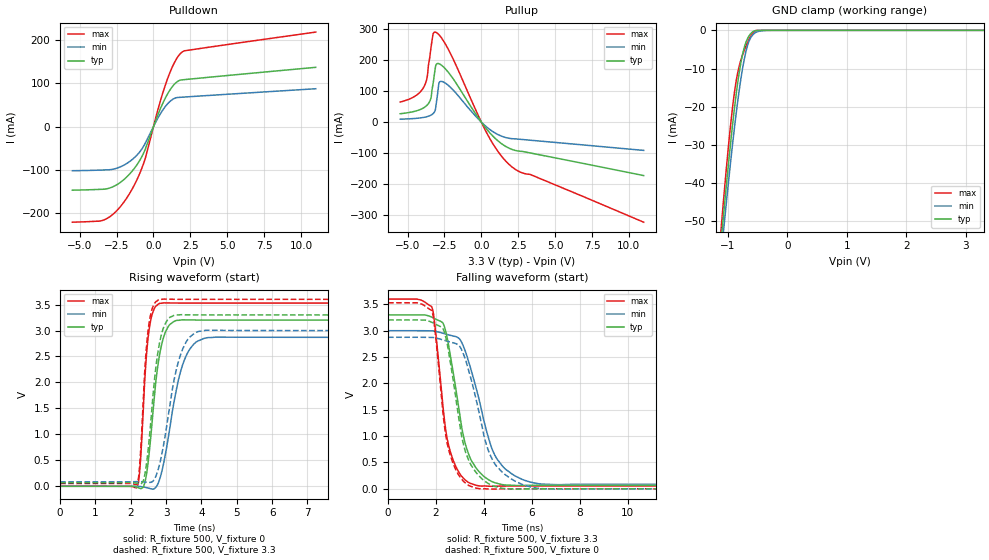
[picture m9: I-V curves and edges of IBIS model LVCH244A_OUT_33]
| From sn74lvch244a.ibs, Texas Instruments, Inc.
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[Model]   LVCH244A_OUT_33
Model_type  3-state
Enable   Active-Low
Vref =   0
Rref =   500
Cref =   50p
Vmeas =   1.5
| variable   typ   min   max
C_comp   4.99pF   4.68pF   5.36pF
| C_pullup   6.79pF   5.44pF   7.57pF
| C_pulldown   5.99pF   4.56pF   7.14pF
| C_tri-state   4.99pF   4.68pF   5.36pF
[Temperature Range]   40   100   -40
| Ambient temperature   25   85   -40
[Voltage range]   3.3   3   3.6
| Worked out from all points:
|   slope of the pulldown table from 0 to 0.495 V, typ, clamps not added: 11.4 ohm
|   slope of the pullup table from 0 to 0.495 V, typ, clamps not added: 16.4 ohm
|   GND clamp passes 1 mA (typ) near -0.62 V on its own axis
|   rising waveform, R_fixture 500, V_fixture 0: 20-80 % time 302ps typ, 479ps min, 190ps max; typ from 0 V to 3.2 V
|   falling waveform, R_fixture 500, V_fixture 3.3: 20-80 % time 767ps typ, 1.07ns min, 558ps max; typ from 3.3 V to 0.068 V
|   rising waveform, R_fixture 500, V_fixture 3.3: 20-80 % time 292ps typ, 464ps min, 185ps max; typ from 0.068 V to 3.3 V
|   falling waveform, R_fixture 500, V_fixture 0: 20-80 % time 739ps typ, 1ns min, 551ps max; typ from 3.2 V to 0 V
[GND Clamp]
| LVCH244A_OUT_33
|   Voltage   I(typ)   I(min)   I(max)
-5.5V     -943.7mA   -897.4mA   -1.02A
-1.13V    -57.95mA   -61.61mA   -54.83mA
-1.1V     -52.83mA   -56.76mA   -49.28mA
-1.075V   -48.62mA   -52.78mA   -44.76mA
-1.05V    -44.49mA   -48.86mA   -40.33mA
-945mV    -28.12mA   -33.13mA   -23.39mA
-845mV    -14.88mA   -19.82mA   -11.9mA
-770mV    -7.53mA    -11.54mA   -7.224mA
-700mV    -3.298mA   -5.769mA   -4.298mA
-630mV    -1.124mA   -2.323mA   -1.902mA
-550mV    -125.2uA   -727.7uA   -227uA
3.3V      1.171nA    103.7nA    -1.528nA
[Pulldown]
| LVCH244A_OUT_33
|   Voltage   I(typ)   I(min)   I(max)
-5.5V     -146.4mA   -101.6mA   -220.3mA
-3.715V   -144.7mA   -100.3mA   -217.9mA
-3.27V    -143.9mA   -99.76mA   -213.7mA
-2.52V    -134.6mA   -96.13mA   -194.9mA
-1.76V    -114.3mA   -83.77mA   -161.9mA
-1.14V    -88.83mA   -66.3mA    -123.8mA
-625mV    -57.63mA   -42.51mA   -80.68mA
390mV     34.91mA    25.18mA    49.89mA
1.01V     78.63mA    54.56mA    115.5mA
1.49V     100.2mA    66.1mA     152mA
1.93V     107.9mA    67.88mA    171.6mA
11V       136.8mA    87.39mA    218mA
[Pullup]
| LVCH244A_OUT_33
|   Voltage   I(typ)   I(min)   I(max)
-5.5V     27.15mA    9.676mA    64.84mA
-4.47V    35.52mA    12.08mA    84.48mA
-3.88V    47.09mA    15.63mA    115mA
-3.675V   55mA       17.9mA     145.1mA
-3.43V    75.88mA    22.33mA    234.3mA
-3.27V    125.3mA    27.62mA    284.1mA
-3.065V   185.7mA    57.97mA    288.8mA
-2.875V   188mA      125.7mA    281.3mA
-2.57V    177.9mA    129.2mA    261.6mA
385mV     -24.04mA   -16.62mA   -36.62mA
1.895V    -84.17mA   -52.11mA   -136.8mA
11V       -171.9mA   -90.86mA   -321.9mA
[Ramp]
| LVCH244A_OUT_33
| variable   typ   min   max
dV/dt_r   1.95/3.12E-10   1.76/5.01E-10   2.14/1.97E-10
dV/dt_f   1.94/7.68E-10   1.75/1.10E-09   2.13/5.60E-10
R_load = 500
[Rising Waveform]
| LVCH244A_OUT_33
R_fixture =   500
C_fixture =   0
L_fixture =   0
V_fixture =   0
V_fixture_min = 0
V_fixture_max = 0
|   Time   V(typ)   V(min)   V(max)
0s        876.5pV    2.906nV    29.23nV
2.175ns   -18.06mV   -1.004mV   -17.43mV
2.26ns    -40.15mV   -4.506mV   367.3mV
2.415ns   123.3mV    -21.91mV   2.255V
2.52ns    639.2mV    -39.66mV   3.022V
2.735ns   2.166V     3.31mV     3.481V
2.92ns    2.852V     410.9mV    3.531V
3.48ns    3.206V     2.365V     3.529V
4.195ns   3.201V     2.864V     3.529V
50ns      3.201V     2.87V      3.529V
[Falling Waveform]
| LVCH244A_OUT_33
R_fixture =   500
C_fixture =   0
L_fixture =   0
V_fixture =   3.3
V_fixture_min = 3
V_fixture_max = 3.6
|   Time   V(typ)   V(min)   V(max)
0s        3.3V       3V         3.6V
1.82ns    3.258V     2.997V     3.455V
2.285ns   3.149V     2.952V     1.597V
2.48ns    2.837V     2.927V     923.5mV
2.8ns     1.982V     2.891V     451.6mV
3.23ns    844.2mV    2.603V     163.6mV
3.78ns    334.8mV    1.732V     56.28mV
4.575ns   100.3mV    548.2mV    49.4mV
6.43ns    67.29mV    88.94mV    52.84mV
50ns      68.11mV    84.28mV    52.74mV
[Rising Waveform]
| LVCH244A_OUT_33
R_fixture =   500
C_fixture =   0
L_fixture =   0
V_fixture =   3.3
V_fixture_min = 3
V_fixture_max = 3.6
|   Time   V(typ)   V(min)   V(max)
0s        68.08mV    84.24mV    52.73mV
2.17ns    60.77mV    89.58mV    43.55mV
2.255ns   47.8mV     89.66mV    439mV
2.4ns     234.7mV    81.26mV    2.277V
2.49ns    692.8mV    75.69mV    3.006V
2.695ns   2.208V     170.9mV    3.545V
2.83ns    2.816V     468.3mV    3.599V
3.42ns    3.304V     2.557V     3.6V
4.135ns   3.3V       3.004V     3.6V
50ns      3.3V       3V         3.6V
[Falling Waveform]
| LVCH244A_OUT_33
R_fixture =   500
C_fixture =   0
L_fixture =   0
V_fixture =   0
V_fixture_min = 0
V_fixture_max = 0
|   Time   V(typ)   V(min)   V(max)
0s        3.203V     2.875V     3.53V
1.82ns    3.16V      2.872V     3.381V
1.955ns   3.129V     2.864V     3.026V
2.285ns   3.045V     2.826V     1.474V
2.58ns    2.458V     2.787V     661.9mV
3.15ns    837.2mV    2.552V     143.3mV
3.775ns   256.7mV    1.497V     3.63mV
4.52ns    36.08mV    432.8mV    -4.613mV
6.4ns     -851.2uV   2.682mV    99.96uV
50ns      25.96uV    43.62uV    7.565uV
